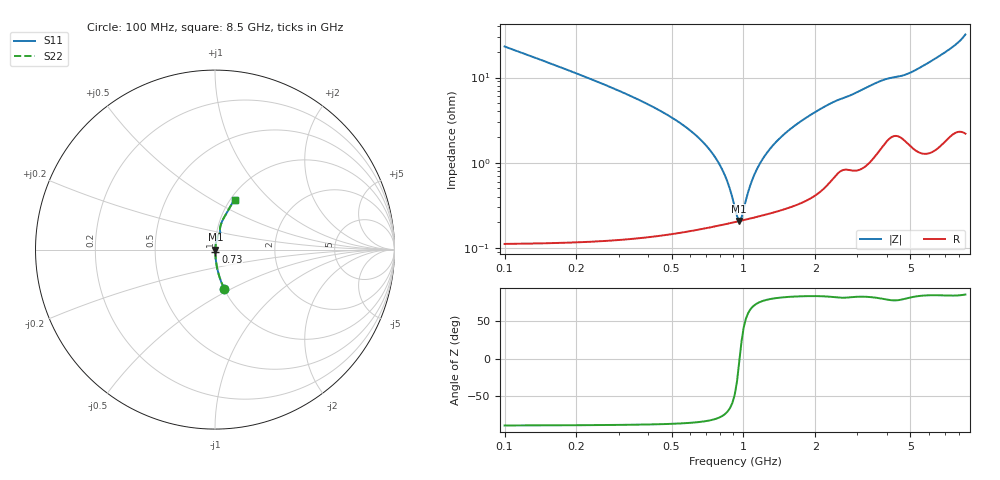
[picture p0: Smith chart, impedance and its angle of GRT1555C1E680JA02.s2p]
!Murata Part Number: GRT1555C1E680JA02
!These Parameters are Measured in Series Mode Connection
!Data Generated on Jun 19, 2026
!  o--ll--o
!Port1  Port2
!  o------o
!Operation Temp=25[degC], DC Bias Voltage=0[V]
!Freq. Start=100[MHz] Stop=9[GHz] 401[Steps]
# Hz S RI R 50
!Freq.(Hz) S11(Real) S11(Imag) S21(Real) S21(Imag) S12(Real) S12(Imag) S22(Real) S22(Imag)
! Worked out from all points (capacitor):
!   401 points, 100 MHz to 8.5 GHz, reference 50 ohm
!   read as one part in series: C = 68.1 pF near 142 MHz
!   lowest |Z| = 207 mohm at 961 MHz (marker M1)
!   series resonance near 963.8 MHz, so ESL is about 400 pH
!   S11 on the Smith chart (normalised r, x): 100 MHz: 1.00, -0.46; 730 MHz: 1.00, -0.03; 8.5 GHz: 1.04, +0.64
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1e8  0.0518 -0.2192  0.9482 0.2192  0.9482 0.2192  0.0518 -0.2192
2.68e8  0.00762 -0.0798  0.9924 0.0798  0.9924 0.0798  0.00762 -0.0798
6.04e8  0.00213 -0.0233  0.9979 0.0233  0.9979 0.0233  0.00213 -0.0233
7.3e8  0.00193 -0.0135  0.9981 0.0135  0.9981 0.0135  0.00193 -0.0135
8.14e8  0.00193 -0.00816  0.9981 0.00816  0.9981 0.00816  0.00193 -0.00816
8.56e8  0.00195 -0.00571  0.998 0.00571  0.998 0.00571  0.00195 -0.00571
9.19e8  0.00201 -0.00229  0.998 0.00229  0.998 0.00229  0.00201 -0.00229
9.61e8  0.00206 -0.000139  0.9979 0.000139  0.9979 0.000139  0.00206 -0.000139
1.003e9  0.00213 0.00192  0.9979 -0.00192  0.9979 -0.00192  0.00213 0.00192
1.066e9  0.00223 0.00485  0.9978 -0.00485  0.9978 -0.00485  0.00223 0.00485
1.108e9  0.00231 0.00672  0.9977 -0.00672  0.9977 -0.00672  0.00231 0.00672
1.192e9  0.00249 0.0103  0.9975 -0.0103  0.9975 -0.0103  0.00249 0.0103
1.318e9  0.00281 0.0153  0.9972 -0.0153  0.9972 -0.0153  0.00281 0.0153
1.507e9  0.00338 0.0223  0.9966 -0.0223  0.9966 -0.0223  0.00338 0.0223
1.78e9  0.00445 0.0316  0.9956 -0.0316  0.9956 -0.0316  0.00445 0.0316
2.116e9  0.00647 0.0426  0.9935 -0.0426  0.9935 -0.0426  0.00647 0.0426
2.914e9  0.0121 0.0632  0.9879 -0.0632  0.9879 -0.0632  0.0121 0.0632
3.67e9  0.0205 0.0849  0.9795 -0.0849  0.9795 -0.0849  0.0205 0.0849
4.3e9  0.0294 0.0941  0.9706 -0.0941  0.9706 -0.0941  0.0294 0.0941
5.707e9  0.0308 0.1329  0.9692 -0.1329  0.9692 -0.1329  0.0308 0.1329
7.114e9  0.0562 0.1891  0.9438 -0.1891  0.9438 -0.1891  0.0562 0.1891
8.5e9  0.1088 0.2789  0.8912 -0.2789  0.8912 -0.2789  0.1088 0.2789
